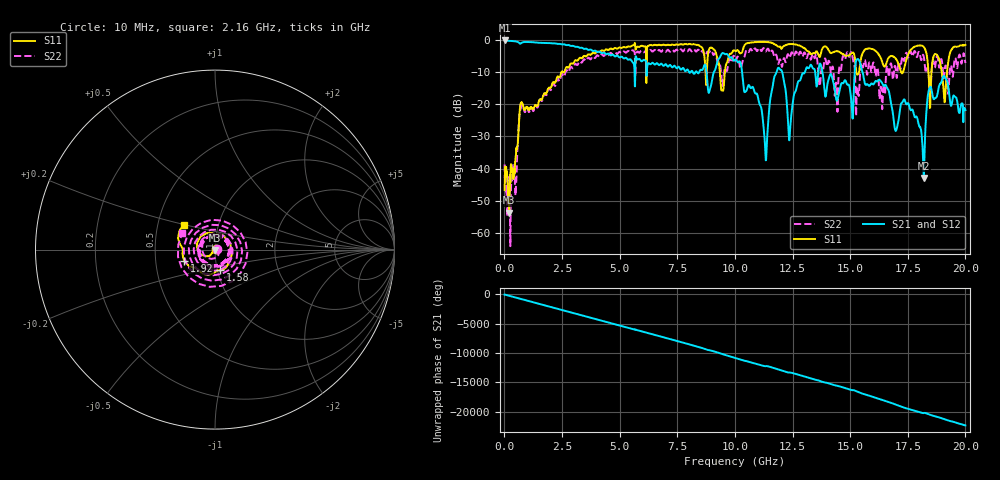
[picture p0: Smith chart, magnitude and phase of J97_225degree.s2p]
!Keysight Technologies,N5222A,MY51421036,A.10.65.16
!Date: Friday, March 31, 2023 15:13:16
!Correction: S11(Full 2 Port(1,2))
!S21(Full 2 Port(1,2))
!S12(Full 2 Port(1,2))
!S22(Full 2 Port(1,2))
!S2P File: Measurements: S11, S21, S12, S22:
# Hz S  dB  R 50
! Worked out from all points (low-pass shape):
!   2000 points, 10 MHz to 20 GHz, reference 50 ohm
!   highest |S21| = -0.08 dB at 10 MHz (marker M1); lowest = -42.9 dB at 18.2 GHz (marker M2)
!   |S21| within 3 dB of the highest: start of sweep to 3.778 GHz
!   lowest |S11| = -53.8 dB at 210 MHz (marker M3), VSWR 1.00, Z = 49.9 - j0.176 ohm
!   |S11| at or under -10 dB: start of sweep to 2.474 GHz; 9.35 GHz to 9.564 GHz (213.8 MHz wide, 2.26 % of centre); 18.97 GHz to 19.2 GHz (226.2 MHz wide, 1.18 % of centre)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
!   |S22| runs from -64.2 to -2.4 dB; largest |S21 - S12| = 0.0093
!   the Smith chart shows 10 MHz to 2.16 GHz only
!   S11 on the Smith chart (normalised r, x): 10 MHz: 1.01, +0.01; 1.58 GHz: 1.03, -0.24; 1.92 GHz: 0.70, -0.09; 2.16 GHz: 0.69, +0.20
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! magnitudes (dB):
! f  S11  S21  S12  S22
! 10 MHz  -46.7  -0.1  0.0  -38.7
! 210 MHz  -53.8  -0.2  -0.2  -42.1
! 730 MHz  -19.5  -0.9  -0.9  -20.7
! 1.58 GHz  -18.5  -0.8  -0.8  -18.5
! 1.92 GHz  -14.8  -0.9  -0.9  -15.1
! 2.16 GHz  -13.2  -1.0  -1.0  -13.8
! 3.35 GHz  -5.6  -2.3  -2.3  -7.0
! 6.68 GHz  -1.4  -7.6  -7.6  -3.2
! 8.91 GHz  -2.5  -15.6  -15.6  -3.6
! 9.46 GHz  -15.4  -4.0  -4.0  -14.2
! 10.01 GHz  -3.3  -6.1  -6.1  -6.0
! 11.33 GHz  -0.5  -36.0  -36.1  -3.5
! 11.82 GHz  -1.7  -9.7  -9.7  -5.0
! 12.38 GHz  -1.2  -29.7  -29.6  -5.5
! 13.34 GHz  -4.3  -8.1  -8.1  -4.9
! 14.39 GHz  -3.4  -18.2  -18.1  -13.2
! 15.34 GHz  -10.7  -5.9  -5.9  -15.7
! 16.67 GHz  -5.4  -15.7  -15.7  -11.1
! 18.2 GHz  -2.1  -42.9  -42.5  -5.3
! 18.43 GHz  -14.3  -15.2  -15.1  -12.7
! 19.05 GHz  -15.0  -11.2  -11.1  -11.7
! 20 GHz  -1.5  -21.8  -21.6  -7.1
